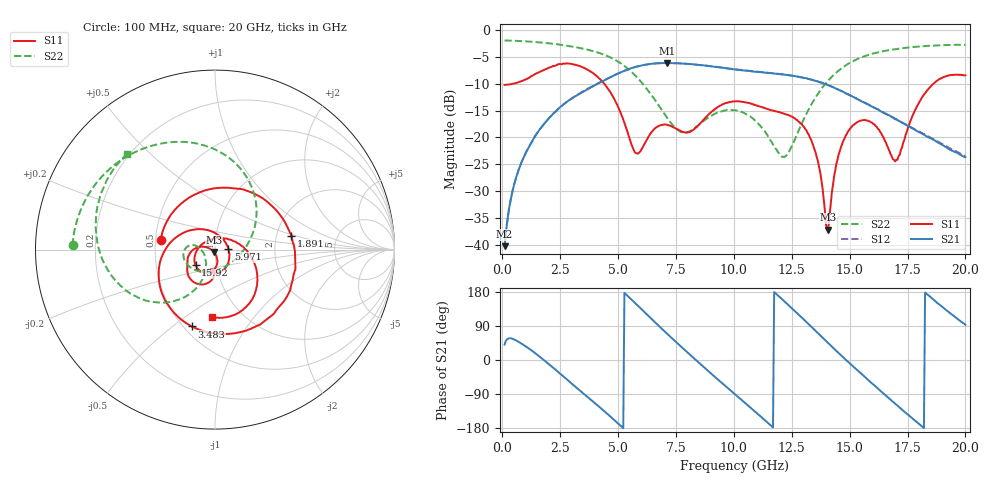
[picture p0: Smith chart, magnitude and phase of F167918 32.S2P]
!  2-Port S-parameters saved by WinCal
! VAR MeasName=S-Parameters (CALIBRATED_DATA) read from VNA (N5242A)
! VAR MeasDate=2016-11-22 10:26:16
! VAR NAME=F167918 32
! VAR FILENAME=F167918 32.S2P
! VAR DATE=2016-11-22 10:26:16
! VAR PHYS_PORTS=1,2
# Hz S DB R 50
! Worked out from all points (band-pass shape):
!   401 points, 100 MHz to 20 GHz, reference 50 ohm
!   highest |S21| = -6.18 dB at 7.115 GHz (marker M1); lowest = -40.2 dB at 100 MHz (marker M2)
!   |S21| within 3 dB of the highest: 4.503 GHz to 13.28 GHz (8.775 GHz wide, 98.7 % of centre)
!   lowest |S11| = -37.1 dB at 14.08 GHz (marker M3), VSWR 1.03, Z = 49.4 - j1.25 ohm
!   |S11| at or under -10 dB: start of sweep to 508.3 MHz; 4.396 GHz to 18.63 GHz (14.23 GHz wide, 124 % of centre)
!   |S22| runs from -23.6 to -2.0 dB; largest |S21 - S12| = 0.0034
!   S11 on the Smith chart (normalised r, x): 100 MHz: 0.53, +0.06; 1.891 GHz: 2.42, +0.46; 3.483 GHz: 0.55, -0.59; 5.971 GHz: 1.16, +0.01; 15.92 GHz: 0.79, -0.14; 20 GHz: 0.73, -0.64
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1e8  -10.24 170.4  -40.18 40.8  -40.10 41.1  -2.00 178.3
6.97e8  -9.77 113.7  -26.13 48.3  -26.09 48.1  -2.09 168.3
1.891e9  -7.27 10.3  -17.04 -4.8  -17.06 -4.8  -2.47 148.3
2.7865e9  -6.25 -58.7  -13.39 -51.1  -13.35 -50.9  -2.97 132.1
3.43325e9  -6.90 -103.5  -11.65 -84.9  -11.58 -84.9  -3.47 119.3
3.483e9  -6.99 -106.7  -11.54 -87.4  -11.46 -87.4  -3.51 118.2
4.92575e9  -13.63 155.4  -8.29 -163.2  -8.27 -163.6  -5.74 81.2
5.9705e9  -22.53 3.3  -6.67 136.6  -6.69 136.3  -9.57 46.0
6.7665e9  -17.86 -75.8  -6.22 89.6  -6.23 89.6  -14.14 13.7
7.11475e9  -17.64 -92.1  -6.18 69.5  -6.19 69.6  -16.31 -4.6
8.458e9  -17.78 -92.1  -6.53 -5.5  -6.51 -5.4  -17.77 -105.3
1.005e10  -13.30 -121.6  -7.37 -90.7  -7.34 -90.6  -14.96 -170.5
1.119425e10  -14.36 -143.9  -7.90 -151.2  -7.87 -151.1  -18.12 168.2
1.21395e10  -15.54 -156.9  -8.33 157.3  -8.31 157.1  -23.59 -157.5
1.338325e10  -21.02 170.5  -9.29 85.5  -9.30 85.6  -13.62 -114.1
1.407975e10  -37.14 -114.2  -10.28 44.5  -10.31 44.5  -9.44 -125.2
1.47265e10  -20.62 -85.5  -11.53 6.8  -11.53 7.2  -6.92 -139.6
1.59205e10  -17.19 -141.3  -14.19 -59.2  -14.15 -58.7  -4.54 -165.4
1.67165e10  -22.52 152.3  -15.90 -101.9  -15.94 -101.4  -3.80 179.9
1.706475e10  -24.14 86.3  -16.79 -120.1  -16.72 -119.9  -3.56 174.0
1.835825e10  -11.22 -31.0  -19.87 172.7  -19.70 173.4  -3.00 154.5
2e10  -8.47 -92.2  -23.66 92.9  -23.45 93.0  -2.80 132.4
